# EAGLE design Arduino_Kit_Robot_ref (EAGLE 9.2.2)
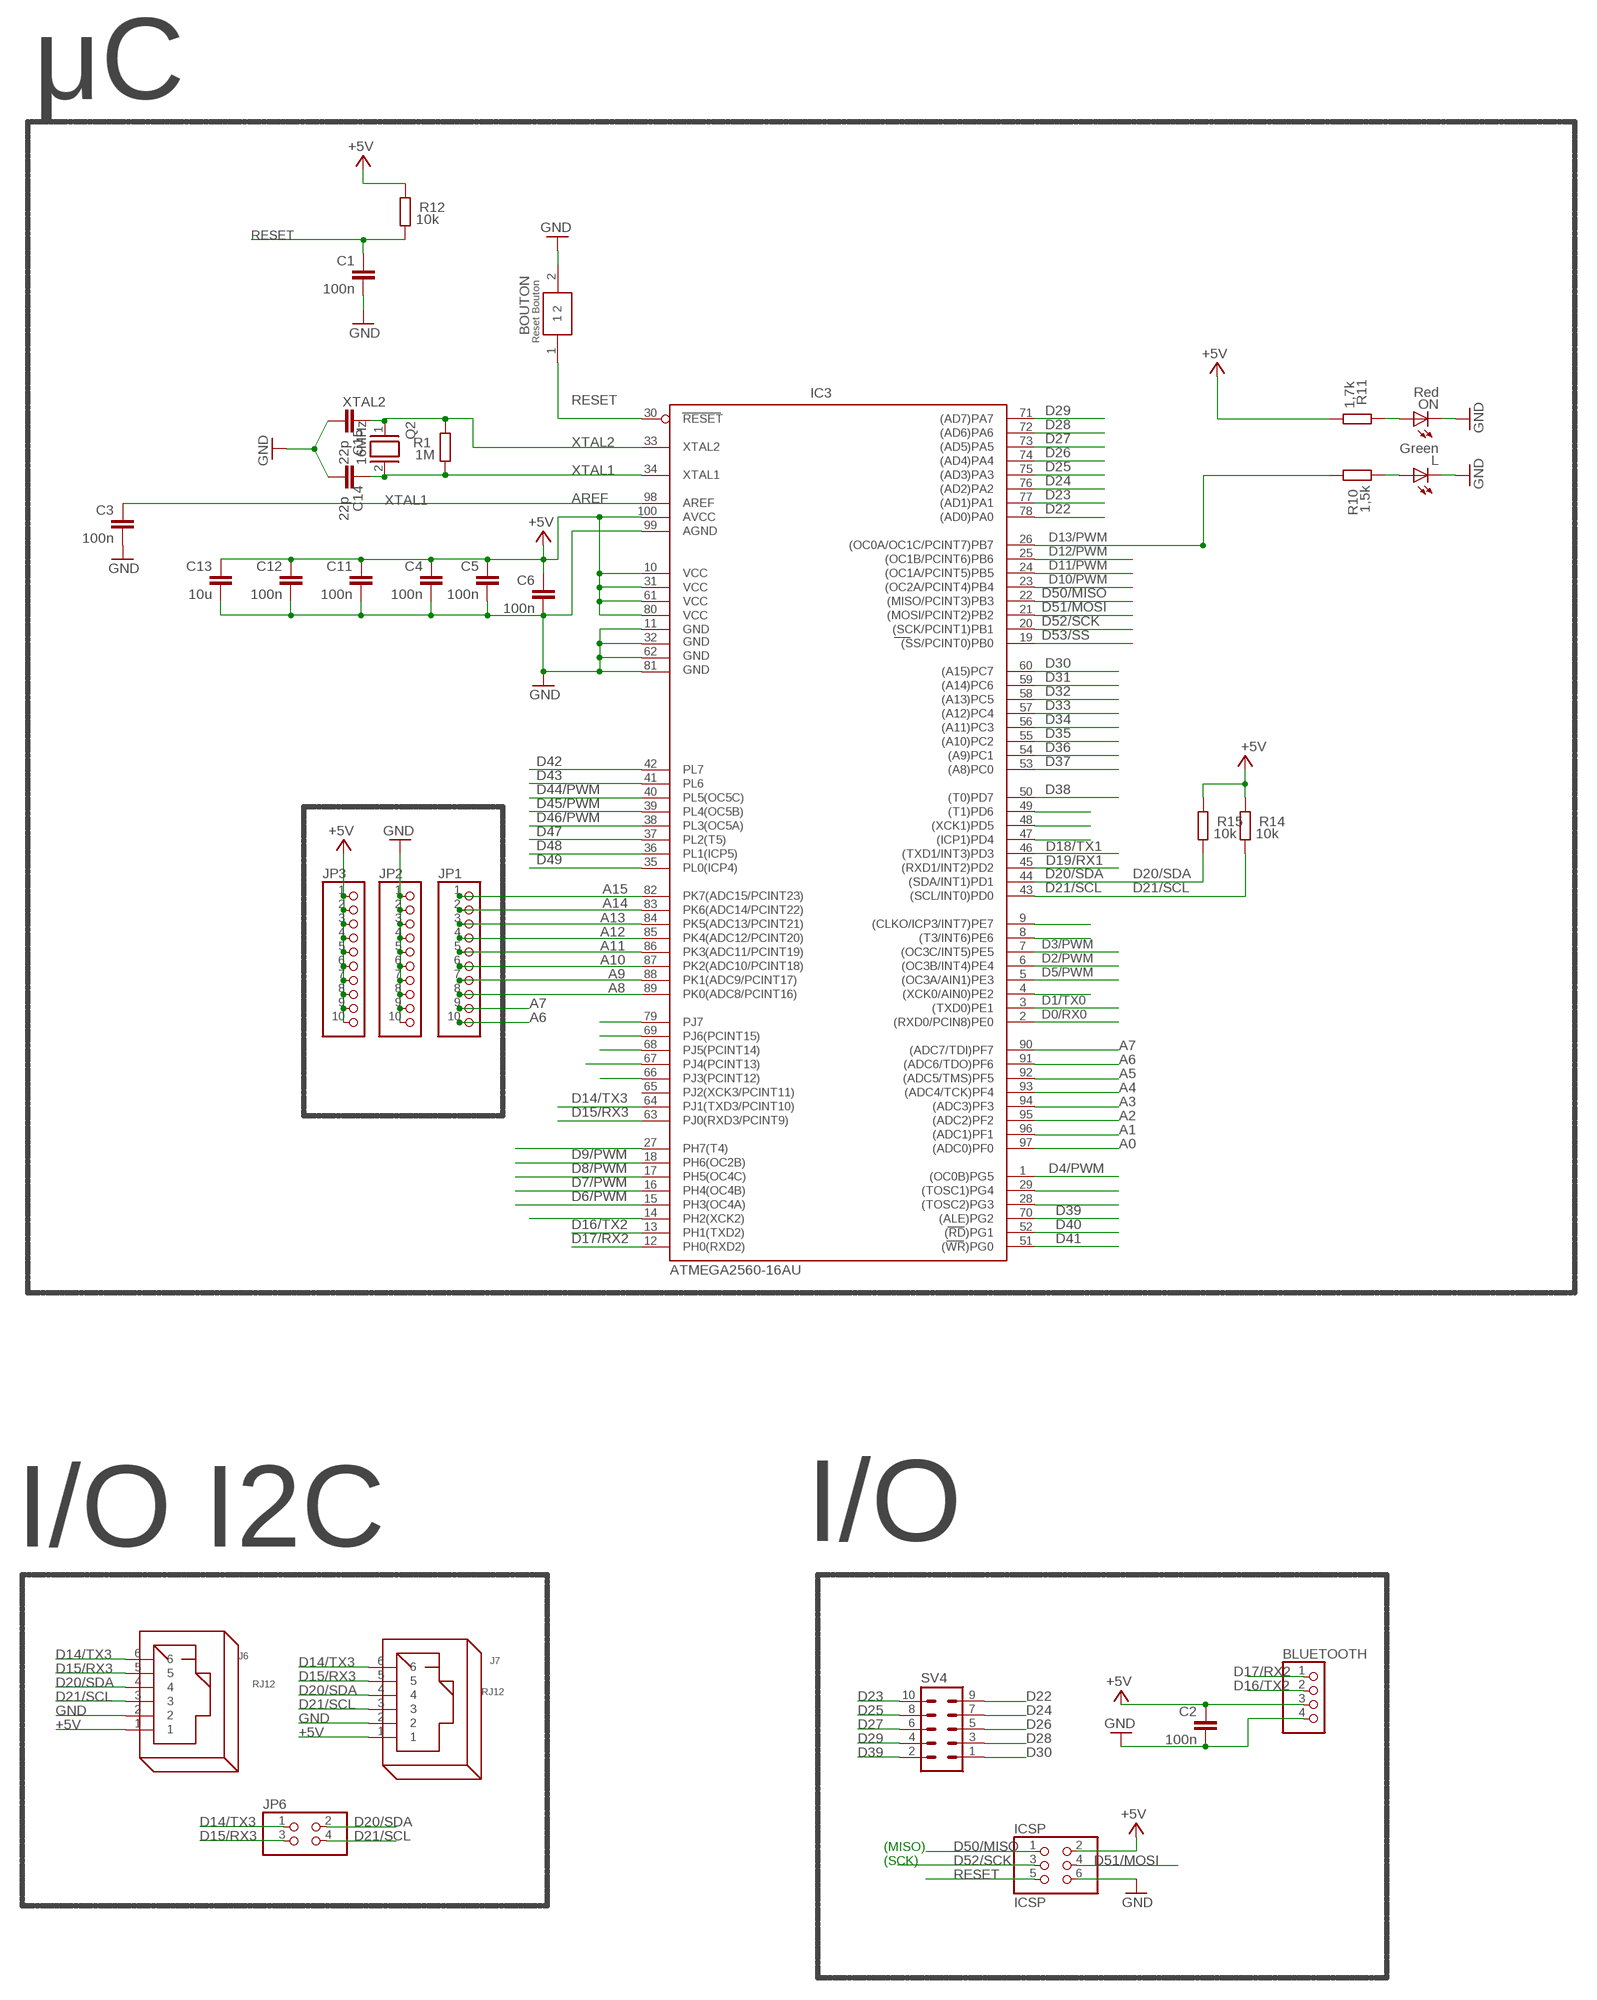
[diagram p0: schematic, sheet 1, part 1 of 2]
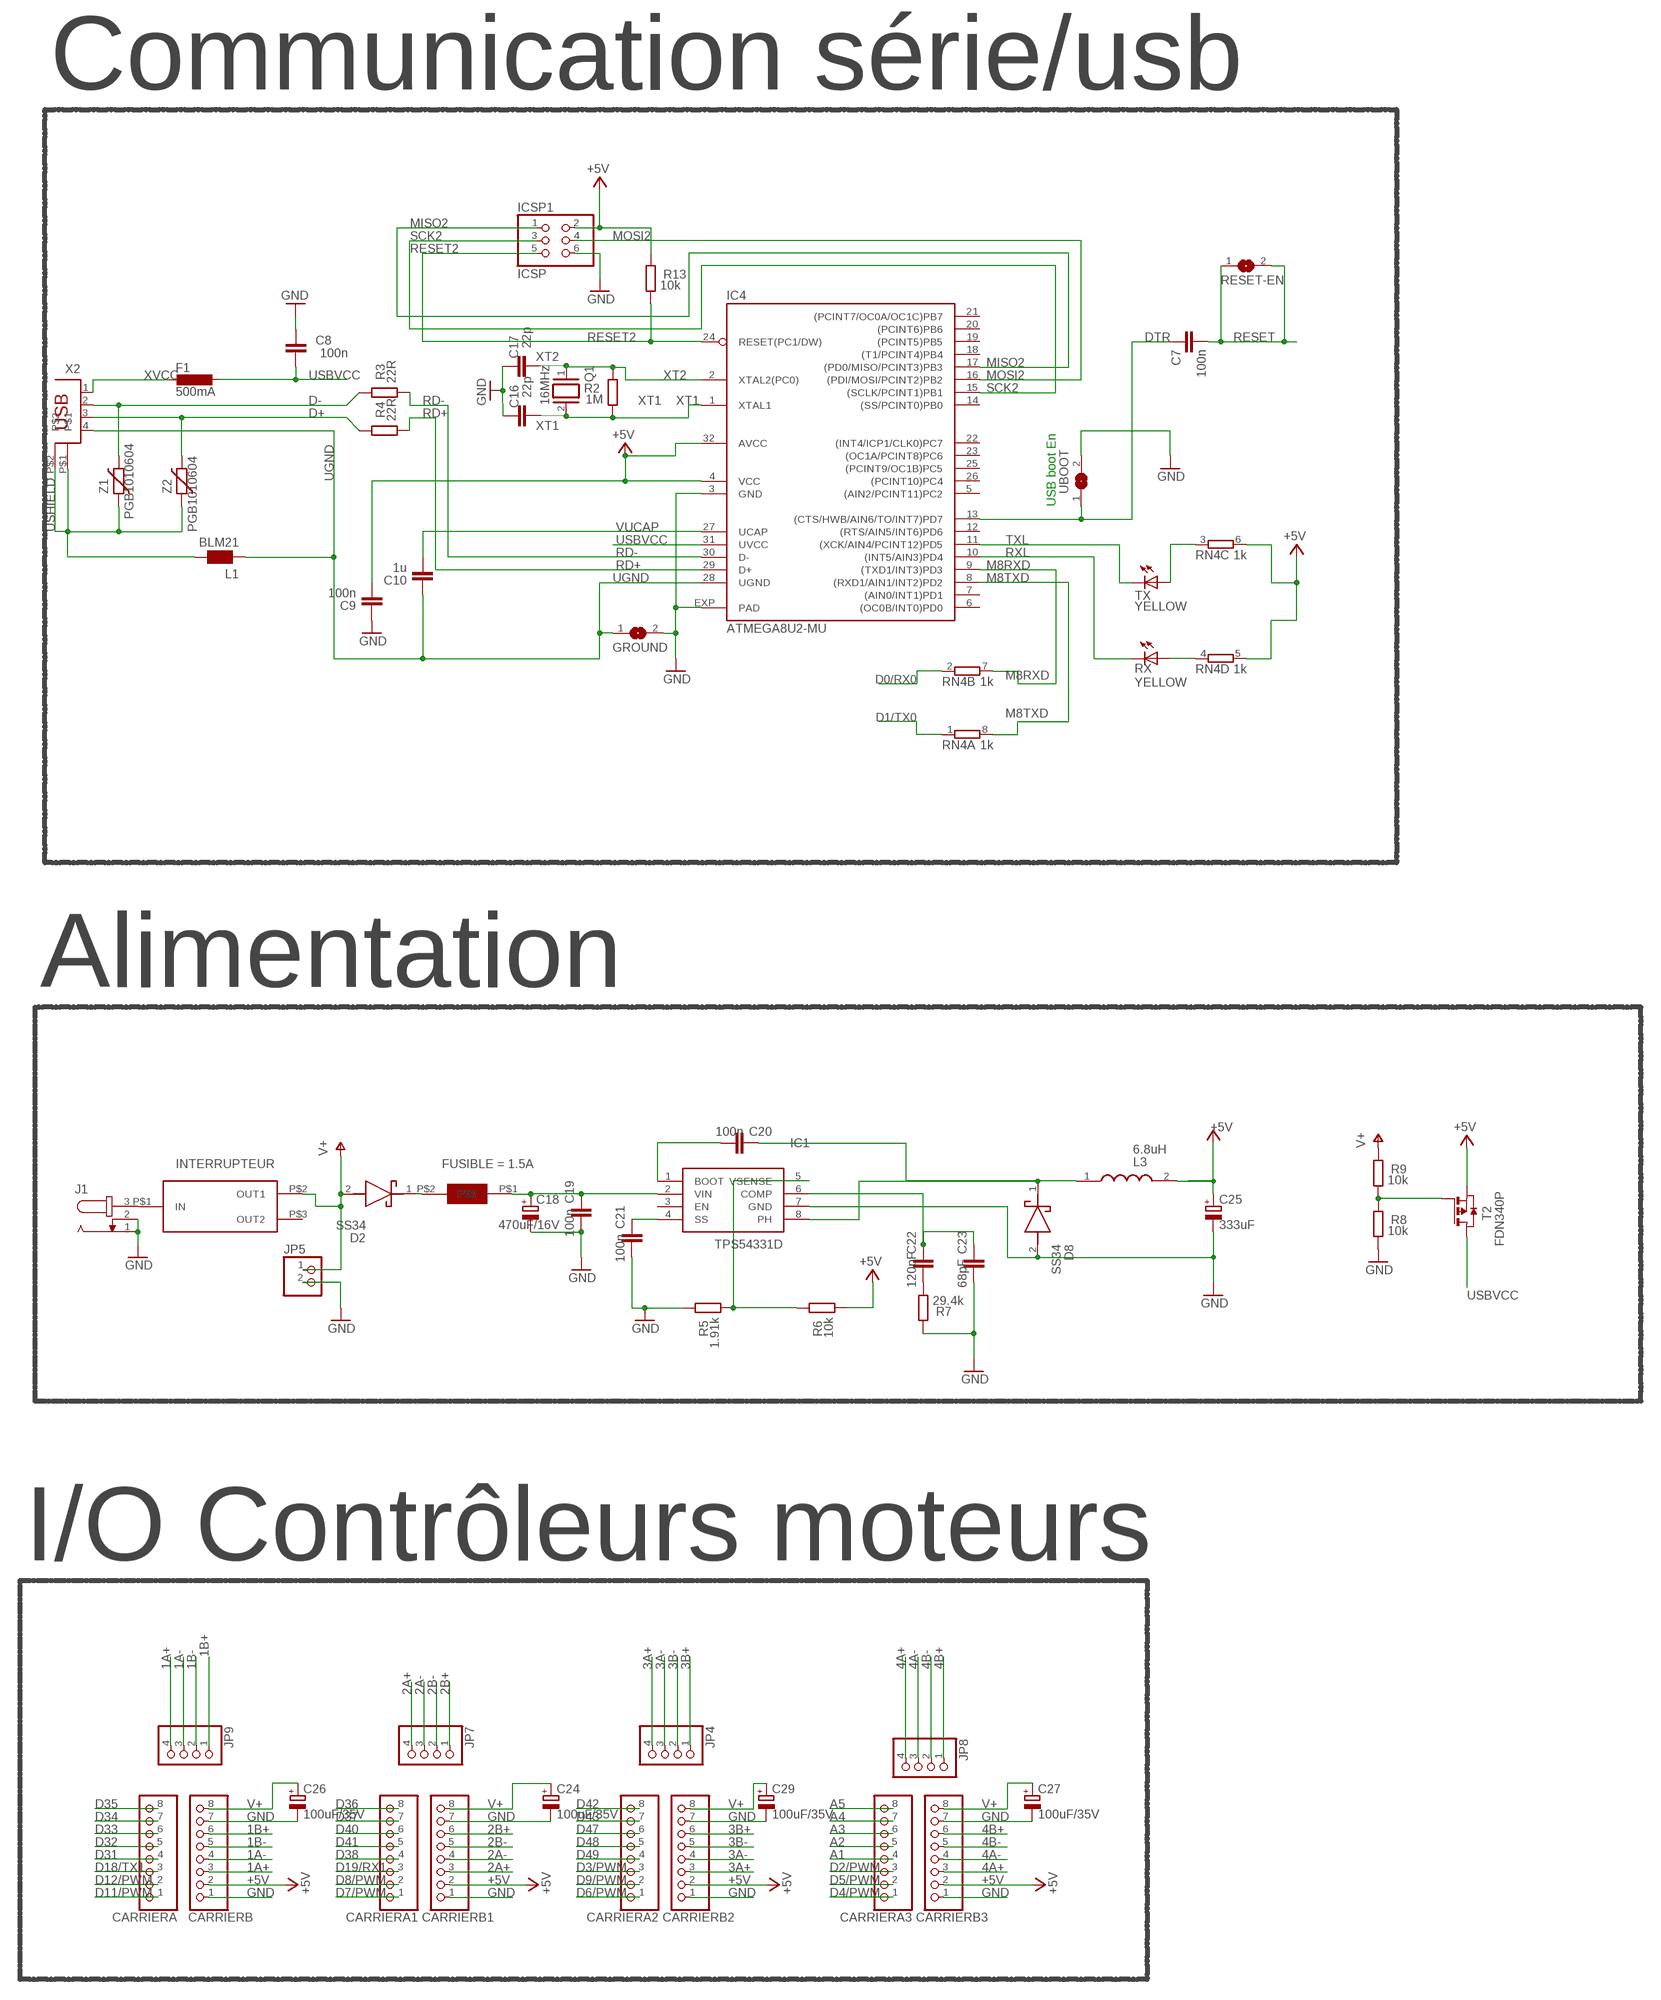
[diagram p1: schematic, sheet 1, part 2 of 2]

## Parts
BLUETOOTH  PINHD-1X4  [1X04]
BOUTON  BOUTON_RESET  [BOUTON_RESET]
C1  100n  C-EU0603-RND  [C0603-ROUND]
C2  100n  C-EU0603-RND  [C0603-ROUND]
C3  100n  C-EU0603-RND  [C0603-ROUND]
C4  100n  C-EU0603-RND  [C0603-ROUND]
C5  100n  C-EU0603-RND  [C0603-ROUND]
C6  100n  C-EU0603-RND  [C0603-ROUND]
C7  100n  C-EU0603-RND  [C0603-ROUND]
C8  100n  C-EUC0603  [C0603]
C9  100n  C-EU0603-RND  [C0603-ROUND]
C10  1u  C-EU0603-RND  [C0603-ROUND]
C11  100n  C-EU0603-RND  [C0603-ROUND]
C12  100n  C-EU0603-RND  [C0603-ROUND]
C13  10u  C-EU0603-RND  [C0603-ROUND]
C14  22p  C-EU0603-RND  [C0603-ROUND]
C15  22p  C-EU0603-RND  [C0603-ROUND]
C16  22p  C-EU0603-RND  [C0603-ROUND]
C17  22p  C-EU0603-RND  [C0603-ROUND]
C18  470uF/16V  CPOL-EUF  [PANASONIC_F]
C19  100n  C-EU0603-RND  [C0603-ROUND]
C20  100n  C-EU0603-RND  [C0603-ROUND]
C21  100n  C-EU0603-RND  [C0603-ROUND]
C22  120pF  C-EU0603-RND  [C0603-ROUND]
C23  68pF  C-EU0603-RND  [C0603-ROUND]
C24  100uF/35V  CPOL-EUF  [PANASONIC_F]
C25  333uF  CPOL-EUD  [PANASONIC_D]
C26  100uF/35V  CPOL-EUF  [PANASONIC_F]
C27  100uF/35V  CPOL-EUF  [PANASONIC_F]
C29  100uF/35V  CPOL-EUF  [PANASONIC_F]
CARRIERA  PINHD-1X8  [1X08]
CARRIERA1  PINHD-1X8  [1X08]
CARRIERA2  PINHD-1X8  [1X08]
CARRIERA3  PINHD-1X8  [1X08]
CARRIERB  PINHD-1X8  [1X08]
CARRIERB1  PINHD-1X8  [1X08]
CARRIERB2  PINHD-1X8  [1X08]
CARRIERB3  PINHD-1X8  [1X08]
D2  SS34  [DIOM8059X256N]
D8  SS34  [DIOM8059X256N]
F1  500mA  L-EUL1812  [L1812]
GROUND  SJ  [SJ]
IC1  TPS54331D  [SOIC127P600X175-8N]
IC3  ATMEGA2560-16AU  ATMEGA1280-16AU  [TQFP100]
IC4  ATMEGA8U2-MU  [QFN32]
ICSP  ICSP  PINHD-2X3  [2X03]
ICSP1  ICSP  PINHD-2X3  [2X03]
J1  JACK-PLUG1  [SPC4078]
J6  RJ12  [RJ12]
J7  RJ12  [RJ12]
JP1  PINHD-1X10  [1X10]
JP2  PINHD-1X10  [1X10]
JP3  PINHD-1X10  [1X10]
JP4  PINHD-1X4/90  [1X04/90]
JP5  PINHD-1X2  [1X02]
JP6  PINHD-2X2  [2X02]
JP7  PINHD-1X4/90  [1X04/90]
JP8  PINHD-1X4/90  [1X04/90]
JP9  PINHD-1X4/90  [1X04/90]
L  Green  LEDCHIP-LED0805  [CHIP-LED0805]
L1  BLM21  WE-CBF_0805  [0805]
L3  6.8uH  7447709006  [WE-PD_1260/1245/1280/121054]
ON  Red  LEDCHIP-LED0805  [CHIP-LED0805]
Q1  16MHz  XTAL/S  [QS]
Q2  16MHz  XTAL/S  [QS]
R1  1M  R-EU_R0603  [R0603-ROUND]
R2  1M  R-EU_R0603  [R0603-ROUND]
R3  22R  R-EU_R0603  [R0603-ROUND]
R4  22R  R-EU_R0603  [R0603-ROUND]
R5  1.91k  R-EU_R0603  [R0603-ROUND]
R6  10k  R-EU_R0603  [R0603-ROUND]
R7  29.4k  R-EU_R0603  [R0603-ROUND]
R8  10k  R-EU_R0603  [R0603-ROUND]
R9  10k  R-EU_R0603  [R0603-ROUND]
R10  1,5k  R-EU_R0603  [R0603-ROUND]
R11  1,7k  R-EU_R0603  [R0603-ROUND]
R12  10k  R-EU_R0603  [R0603-ROUND]
R13  10k  R-EU_R0603  [R0603-ROUND]
R14  10k  R-EU_R0603  [R0603-ROUND]
R15  10k  R-EU_R0603  [R0603-ROUND]
RESET-EN  SJ  [SJ]
RN4  1k  4R-NCAY16  [CAY16]
RX  YELLOW  LEDCHIP-LED0805  [CHIP-LED0805]
SV4  MA05-2  [MA05-2]
T2  FDN340P  PMOSSOT23  [SOT-23]
TX  YELLOW  LEDCHIP-LED0805  [CHIP-LED0805]
U$2  SMD-150  [SMDF-150]
U$3  INTERRUPT  [INTERRUPTEUR]
UBOOT  SJ  [SJ]
X2  PN61729  [PN61729]
Z1  PGB1010604  VARISTORCN0603  [CT/CN0603]
Z2  PGB1010604  VARISTORCN0603  [CT/CN0603]

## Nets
1A+: CARRIERB.3 JP9.4
1A-: CARRIERB.4 JP9.3
1B+: CARRIERB.6 JP9.1
1B-: CARRIERB.5 JP9.2
2A+: CARRIERB1.3 JP7.4
2A-: CARRIERB1.4 JP7.3
2B+: CARRIERB1.6 JP7.1
2B-: CARRIERB1.5 JP7.2
3A+: CARRIERB2.3 JP4.4
3A-: CARRIERB2.4 JP4.3
3B+: CARRIERB2.6 JP4.1
3B-: CARRIERB2.5 JP4.2
4A+: CARRIERB3.3 JP8.4
4A-: CARRIERB3.4 JP8.3
4B+: CARRIERB3.6 JP8.1
4B-: CARRIERB3.5 JP8.2
+5V: BLUETOOTH.3 C2.1 C4.1 C5.1 C6.1 C9.1 C11.1 C12.1 C13.1 C25.+ CARRIERB1.2 CARRIERB2.2 CARRIERB3.2 CARRIERB.2 IC3.10(VCC) IC3.31(VCC1) IC3.61(VCC2) IC3.80(VCC3) IC3.100(AVCC) IC4.4(VCC) IC4.32(AVCC) ICSP1.2 ICSP.2 J6.1 J7.1 JP3.1 JP3.2 JP3.3 JP3.4 JP3.5 JP3.6 JP3.7 JP3.8 JP3.9 JP3.10 L3.2 R6.1 R11.1 R12.2 R13.2 R14.2 R15.2 RN4.5 RN4.6 T2.2(S)
A0: IC3.97((ADC0)PF0)
A1: CARRIERA3.4 IC3.96((ADC1)PF1)
A2: CARRIERA3.5 IC3.95((ADC2)PF2)
A3: CARRIERA3.6 IC3.94((ADC3)PF3)
A4: CARRIERA3.7 IC3.93((ADC4/TCK)PF4)
A5: CARRIERA3.8 IC3.92((ADC5/TMS)PF5)
A6: IC3.91((ADC6/TDO)PF6) JP1.10
A7: IC3.90((ADC7/TDI)PF7) JP1.9
A8: IC3.89(PK0(ADC8/PCINT16)) JP1.8
A9: IC3.88(PK1(ADC9/PCINT17)) JP1.7
A10: IC3.87(PK2(ADC10/PCINT18)) JP1.6
A11: IC3.86(PK3(ADC11/PCINT19)) JP1.5
A12: IC3.85(PK4(ADC12/PCINT20)) JP1.4
A13: IC3.84(PK5(ADC13/PCINT21)) JP1.3
A14: IC3.83(PK6(ADC14/PCINT22)) JP1.2
A15: IC3.82(PK7(ADC15/PCINT23)) JP1.1
AREF: C3.1 IC3.98(AREF)
D0/RX0: IC3.2((RXD0/PCIN8)PE0) RN4.2
D1/TX0: IC3.3((TXD0)PE1) RN4.1
D2/PWM: CARRIERA3.3 IC3.6((OC3B/INT4)PE4)
D3/PWM: CARRIERA2.3 IC3.7((OC3C/INT5)PE5)
D4/PWM: CARRIERA3.1 IC3.1((OC0B)PG5)
D5/PWM: CARRIERA3.2 IC3.5((OC3A/AIN1)PE3)
D6/PWM: CARRIERA2.1 IC3.15(PH3(OC4A))
D7/PWM: CARRIERA1.1 IC3.16(PH4(OC4B))
D8/PWM: CARRIERA1.2 IC3.17(PH5(OC4C))
D9/PWM: CARRIERA2.2 IC3.18(PH6(OC2B))
D10/PWM: IC3.23((OC2A/PCINT4)PB4)
D11/PWM: CARRIERA.1 IC3.24((OC1A/PCINT5)PB5)
D12/PWM: CARRIERA.2 IC3.25((OC1B/PCINT6)PB6)
D13/PWM: IC3.26((OC0A/OC1C/PCINT7)PB7) R10.2
D14/TX3: IC3.64(PJ1(TXD3/PCINT10)) J6.6 J7.6 JP6.1
D15/RX3: IC3.63(PJ0(RXD3/PCINT9)) J6.5 J7.5 JP6.3
D16/TX2: BLUETOOTH.2 IC3.13(PH1(TXD2))
D17/RX2: BLUETOOTH.1 IC3.12(PH0(RXD2))
D18/TX1: CARRIERA.3 IC3.46((TXD1/INT3)PD3)
D19/RX1: CARRIERA1.3 IC3.45((RXD1/INT2)PD2)
D20/SDA: IC3.44((SDA/INT1)PD1) J6.4 J7.4 JP6.2 R15.1
D21/SCL: IC3.43((SCL/INT0)PD0) J6.3 J7.3 JP6.4 R14.1
D22: IC3.78((AD0)PA0) SV4.9
D23: IC3.77((AD1)PA1) SV4.10
D24: IC3.76((AD2)PA2) SV4.7
D25: IC3.75((AD3)PA3) SV4.8
D26: IC3.74((AD4)PA4) SV4.5
D27: IC3.73((AD5)PA5) SV4.6
D28: IC3.72((AD6)PA6) SV4.3
D29: IC3.71((AD7)PA7) SV4.4
D30: IC3.60((A15)PC7) SV4.1
D31: CARRIERA.4 IC3.59((A14)PC6)
D32: CARRIERA.5 IC3.58((A13)PC5)
D33: CARRIERA.6 IC3.57((A12)PC4)
D34: CARRIERA.7 IC3.56((A11)PC3)
D35: CARRIERA.8 IC3.55((A10)PC2)
D36: CARRIERA1.8 IC3.54((A9)PC1)
D37: CARRIERA1.7 IC3.53((A8)PC0)
D38: CARRIERA1.4 IC3.50((T0)PD7)
D39: IC3.70((ALE)PG2) SV4.2
D40: CARRIERA1.6 IC3.52((RD)PG1)
D41: CARRIERA1.5 IC3.51((WR)PG0)
D42: CARRIERA2.8 IC3.42(PL7)
D43: CARRIERA2.7 IC3.41(PL6)
D44/PWM: IC3.40(PL5(OC5C))
D45/PWM: IC3.39(PL4(OC5B))
D46/PWM: IC3.38(PL3(OC5A))
D47: CARRIERA2.6 IC3.37(PL2(T5))
D48: CARRIERA2.5 IC3.36(PL1(ICP5))
D49: CARRIERA2.4 IC3.35(PL0(ICP4))
D50/MISO: IC3.22((MISO/PCINT3)PB3) ICSP.1
D51/MOSI: IC3.21((MOSI/PCINT2)PB2) ICSP.4
D52/SCK: IC3.20((SCK/PCINT1)PB1) ICSP.3
D53/SS: IC3.19((SS/PCINT0)PB0)
D+: R4.2 X2.3 Z2.2
D-: R3.2 X2.2 Z1.2
DTR: C7.1 IC4.13((CTS/HWB/AIN6/TO/INT7)PD7) UBOOT.1
GND: BLUETOOTH.4 BOUTON.2 C1.2 C2.2 C3.2 C4.2 C5.2 C6.2 C8.2 C9.2 C11.2 C12.2 C13.2 C14.1 C15.1 C16.2 C17.2 C18.- C19.1 C21.1 C23.1 C24.- C25.- C26.- C27.- C29.- CARRIERB1.1 CARRIERB1.7 CARRIERB2.1 CARRIERB2.7 CARRIERB3.1 CARRIERB3.7 CARRIERB.1 CARRIERB.7 D8.2(A) GROUND.2 IC1.7(GND) IC3.11(GND) IC3.32(GND1) IC3.62(GND2) IC3.81(GND3) IC3.99(AGND) IC4.3(GND) IC4.EXP(PAD) ICSP1.6 ICSP.6 J1.1 J1.2 J6.2 J7.2 JP2.1 JP2.2 JP2.3 JP2.4 JP2.5 JP2.6 JP2.7 JP2.8 JP2.9 JP2.10 JP5.2 L.C ON.C R5.2 R7.2 R8.1 UBOOT.2
M8RXD: IC4.9((TXD1/INT3)PD3) RN4.7
M8TXD: IC4.8((RXD1/AIN1/INT2)PD2) RN4.8
MISO2: IC4.17((PD0/MISO/PCINT3)PB3) ICSP1.1
MOSI2: IC4.16((PDI/MOSI/PCINT2)PB2) ICSP1.4
N$1: J1.3 U$3.P$1(IN)
N$2: L.A R10.1
N$3: ON.A R11.2
N$4: D2.1(K) U$2.P$2
N$5: C18.+ C19.2 IC1.2(VIN) U$2.P$1
N$6: C20.1 IC1.1(BOOT)
N$7: R8.2 R9.1 T2.3(G)
N$8: C21.2 IC1.4(SS)
N$9: C22.1 R7.1
N$10: IC1.5(VSENSE) R5.1 R6.2
N$11: IC3.49((T1)PD6)
N$12: C22.2 C23.2 IC1.6(COMP)
N$13: C20.2 D8.1(K) IC1.8(PH) L3.1
N$14: IC3.48((XCK1)PD5)
N$15: IC3.47((ICP1)PD4)
N$16: IC3.4((XCK0/AIN0)PE2)
N$17: IC3.9((CLKO/ICP3/INT7)PE7)
N$18: IC3.8((T3/INT6)PE6)
N$19: IC3.29((TOSC1)PG4)
N$20: IC3.28((TOSC2)PG3)
N$21: IC3.27(PH7(T4))
N$22: IC3.14(PH2(XCK2))
N$23: IC3.79(PJ7)
N$24: IC3.69(PJ6(PCINT15))
N$25: IC3.68(PJ5(PCINT14))
N$26: IC3.67(PJ4(PCINT13))
N$27: IC3.66(PJ3(PCINT12))
N$54: RN4.4 RX.A
N$55: RN4.3 TX.A
RD+: IC4.29(D+) R4.1
RD-: IC4.30(D-) R3.1
RESET: BOUTON.1 C1.1 C7.2 IC3.30(RESET) ICSP.5 R12.1 RESET-EN.1 RESET-EN.2
RESET2: IC4.24(RESET(PC1/DW)) ICSP1.5 R13.1
RXL: IC4.10((INT5/AIN3)PD4) RX.C
SCK2: IC4.15((SCLK/PCINT1)PB1) ICSP1.3
TXL: IC4.11((XCK/AIN4/PCINT12)PD5) TX.C
UGND: C10.2 GROUND.1 IC4.28(UGND) L1.1 X2.4
USBVCC: C8.1 F1.1 IC4.31(UVCC) T2.1(D)
USHIELD: L1.2 X2.P$1 X2.P$2 Z1.1 Z2.1
V+: C24.+ C26.+ C27.+ C29.+ CARRIERB1.8 CARRIERB2.8 CARRIERB3.8 CARRIERB.8 D2.2(A) JP5.1 R9.2 U$3.P$2(OUT1)
VUCAP: C10.1 IC4.27(UCAP)
XT1: C16.1 IC4.1(XTAL1) Q1.2 R2.1
XT2: C17.1 IC4.2(XTAL2(PC0)) Q1.1 R2.2
XTAL1: C14.2 IC3.34(XTAL1) Q2.2 R1.1
XTAL2: C15.2 IC3.33(XTAL2) Q2.1 R1.2
XVCC: F1.2 X2.1
Unconnected: IC1.3(EN) IC3.65(PJ2(XCK3/PCINT11)) IC4.5((AIN2/PCINT11)PC2) IC4.6((OC0B/INT0)PD0) IC4.7((AIN0/INT1)PD1) IC4.12((RTS/AIN5/INT6)PD6) IC4.14((SS/PCINT0)PB0) IC4.18((T1/PCINT4)PB4) IC4.19((PCINT5)PB5) IC4.20((PCINT6)PB6) IC4.21((PCINT7/OC0A/OC1C)PB7) IC4.22((INT4/ICP1/CLK0)PC7) IC4.23((OC1A/PCINT8)PC6) IC4.25((PCINT9/OC1B)PC5) IC4.26((PCINT10)PC4) U$3.P$3(OUT2)

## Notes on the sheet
- μC | Communication série/usb
- USB boot En
- Alimentation
- I/O I2C | I/O
- I/O Contrôleurs moteurs
- (MISO)
- (SCK)

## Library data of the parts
BLUETOOTH JP4 JP7-JP9 = pinhead:PINHD-1X4: PIN HEADER
BOUTON = MyLib:BOUTON_RESET
C1-C7 C9-C17 C19-C23 = SmartPrj:C-EU: CAPACITOR, European symbol
C8 = rcl:C-EU: CAPACITOR, European symbol
C18 C24-C27 C29 = rcl:CPOL-EU: POLARIZED CAPACITOR, European symbol; SPICEPREFIX: C
CARRIERA CARRIERA1-CARRIERA3 CARRIERB CARRIERB1-CARRIERB3 = pinhead:PINHD-1X8: PIN HEADER
D2 D8 = SamacSys_Parts:SS34: ON Semi SS34 SMT Schottky Diode, 40V 3A, 2-Pin DO-214AB; DESCRIPTION: ON Semi SS34 SMT Schottky Diode, 40V 3A, 2-Pin DO-214AB; HEIGHT: 2.56mm; MANUFACTURER_NAME: ON Semiconductor; MANUFACTURER_PART_NUMBER: SS34; RS_PART_NUMBER: 1662321
F1 = rcl:L-EU: INDUCTOR, European symbol
GROUND RESET-EN UBOOT = jumper:SJ: SMD solder JUMPER
IC1 = SamacSys_Parts:TPS54331D: Texas Instruments, TPS54331D Step-Down Switching Regulator 3A Adjustable, Minimum of 0.8 V, 8-Pin SOIC Source: Datasheet; DESCRIPTION: Texas Instruments, TPS54331D Step-Down Switching Regulator 3A Adjustable, Minimum of 0.8 V, 8-Pin SOIC; HEIGHT: mm; MANUFACTURER_NAME: Texas Instruments; MANUFACTURER_PART_NUMBER: TPS54331D; RS_PART_NUMBER: 6618521P; RS_PRICE-STOCK: http://uk.rs-online.com/web/p/products/6618521P
IC3 = atmel-2005:ATMEGA*: MICROCONTROLLER 64/128/256 Kbytes FLASH 4 Kbytes EEPROM 8 Kbytes SRAM 86 General Purpose I/O pins 12-channels16-bit PWM 4 x Serial USARTs 16-channels 10-bit A/D
IC4 = atmel:ATMEGA8U2-MU
ICSP ICSP1 = pinhead:PINHD-2X3: PIN HEADER
J1 = con-jack:JACK-PLUG: DC POWER JACK Power Jack, DC, Right Angle, Through Hole, Rated 5A at 16VDC, PC Terminals Distributor: Farnell (www.Farnell.de) Drawing: 84N1161.pdf / 84N1162.pdf Manufacturer: SPC Technology (www.spctechnology.com) Type: SPC4077 / SPC 4078; OC_FARNELL: unknown; OC_NEWARK: unknown
J6 J7 = con-rj:RJ12: RJ12, RJ14 and RJ25 RJ12, RJ14 and RJ25 jacks side mounted http://www.tycoelectronics.com
JP1-JP3 = pinhead:PINHD-1X10: PIN HEADER
JP5 = pinhead:PINHD-1X2: PIN HEADER
JP6 = pinhead:PINHD-2X2: PIN HEADER
L ON RX TX = led:LED: LED
L1 = wuerth-elektronik:WE-CBF: SMD EMI Suppression Ferrite Beads
L3 = SamacSys_Parts:7447709006: Wurth WE-PD Series Shielded Wire-wound SMD Inductor 6.8 uH +/-20% 8.4A Idc; DESCRIPTION: Wurth WE-PD Series Shielded Wire-wound SMD Inductor 6.8 uH +/-20% 8.4A Idc; HEIGHT: mm; MANUFACTURER_NAME: Wurth Elektronik; MANUFACTURER_PART_NUMBER: 7447709006; RS_PART_NUMBER: 7896776; RS_PRICE-STOCK: http://uk.rs-online.com/web/p/products/7896776
Q1 Q2 = special:XTAL/S: CRYSTAL
R1-R15 = SmartPrj:R-EU_: RESISTOR, European symbol
RN4 = resistor-dil:4R-N: Array Chip Resistor Source: RS Component / Phycomp
SV4 = con-lstb:MA05-2: PIN HEADER; OC_FARNELL: unknown; OC_NEWARK: unknown
T2 = zetex:PMOSSOT23: MOS FET
U$2 = MyLib:SMD-150; FUSIBLE: 1.5A
U$3 = MyLib:INTERRUPT
X2 = SmartPrj:PN61729: BERG USB connector
Z1 Z2 = varistor:VARISTOR: VARISTOR

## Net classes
0 default: width 0.15 mm, drill 0.3 mm, clearance 0.15 mm

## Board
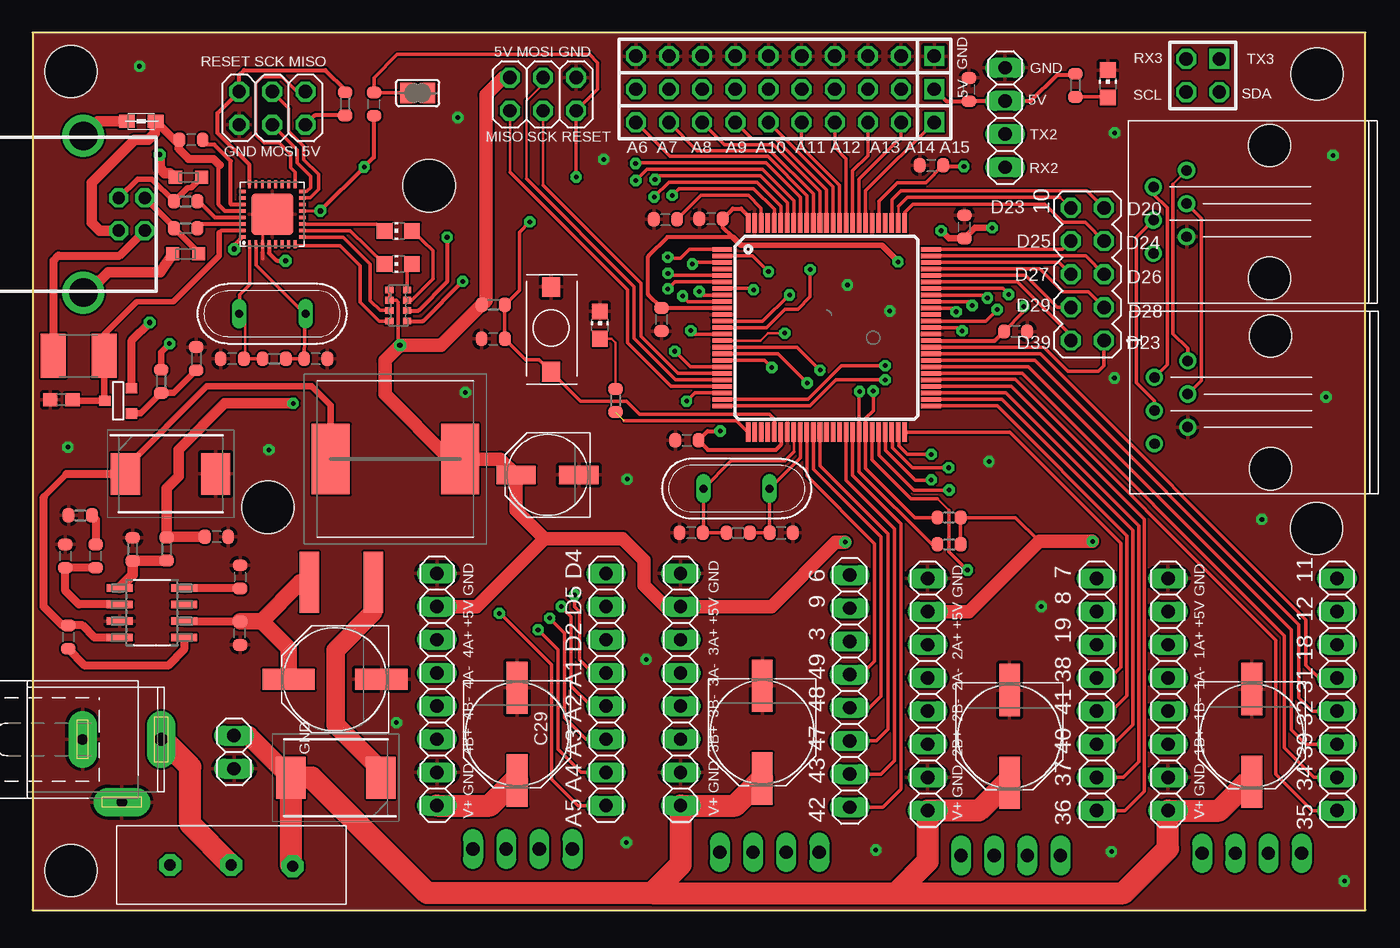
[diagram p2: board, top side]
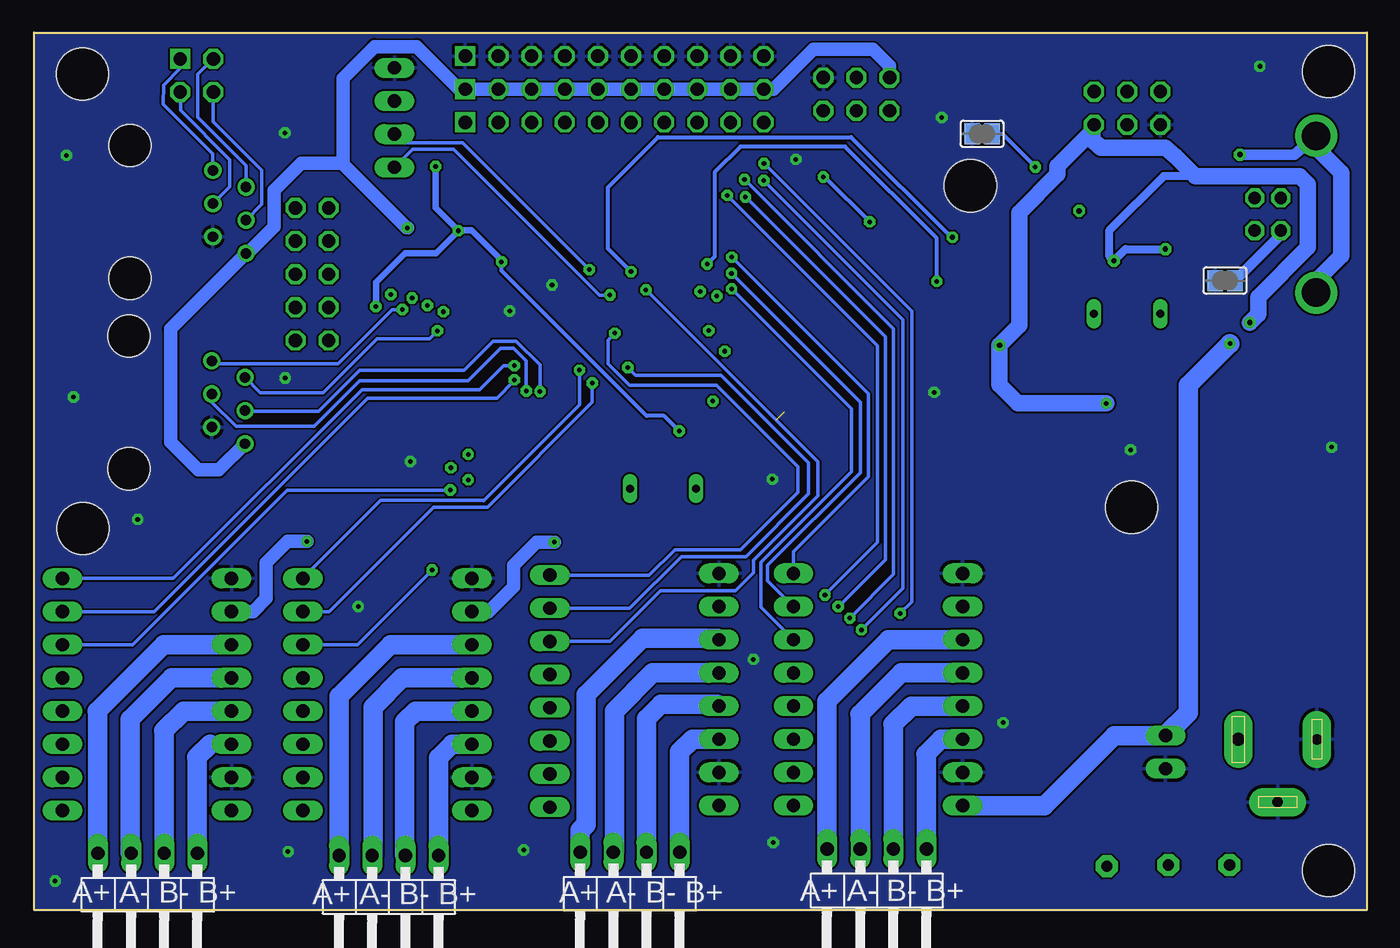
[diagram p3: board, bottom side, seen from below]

Size 102.1 x 67.2 mm. Coordinates in mm from the lower left corner, seen from the top.
Outline: 102.1,0 102.1,67.2 0,67.2 0,0 102.1,0
Copper layers (1*16): Top 0.035mm / dielectric 1.5mm / Bottom 0.035mm
Design rules "default *": minimum track width 0.15mm, minimum drill 0.3mm, track to track 0.15mm, track to pad 0.15mm, pad to pad 0.15mm, via to via 0.15mm, smd to smd 0.15mm, copper to edge 0mil, drill to drill 0.3mm, minimum pad ring 10mil, minimum via ring 10mil, stop-mask expansion 2mil, vias tented up to drill 1mil, thermal gap 10mil
Holes 4 mm at 18.02,30.85 30.38,55.48 2.93,64.23 2.95,3.02 98.35,29.22 98.4,64.03

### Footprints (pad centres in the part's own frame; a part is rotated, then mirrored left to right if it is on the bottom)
1X04 = drill 1.016 long: 1 -3.81,0; 2 -1.27,0; 3 1.27,0; 4 3.81,0
BOUTON_RESET = smd 1.5 x 1.4: 1 0.752,0.7; 2 7.249,0.702
C0603-ROUND = smd 0.898 x 1.1: 1 -0.889,0; 2 0.889,0
C0603 = smd 1.1 x 1: 1 -0.85,0; 2 0.85,0
PANASONIC_F = smd 4 x 1.6: + 3.55,0; - -3.55,0
PANASONIC_D = smd 3 x 1.4: + 2.4,0; - -2.4,0
1X08 = drill 1.016 long: 1 -8.89,0; 2 -6.35,0; 3 -3.81,0; 4 -1.27,0; 5 1.27,0; 6 3.81,0; 7 6.35,0; 8 8.89,0
DIOM8059X256N = smd 2.25 x 3.2: 1 -3.45,0; 2 3.45,0
L1812 = smd 1.9 x 3.4: 1 -1.95,0; 2 1.95,0
SJ = smd 1.168 x 1.6: 1 -0.762,0; 2 0.762,0
SOIC127P600X175-8N = smd 1.981 x 0.559: 1 -2.464,1.905; 2 -2.464,0.635; 3 -2.464,-0.635; 4 -2.464,-1.905; 5 2.464,-1.905; 6 2.464,-0.635; 7 2.464,0.635; 8 2.464,1.905
TQFP100 = smd 1.5 x 0.35: 1 -8,6; 2 -8,5.5; 3 -8,5; 4 -8,4.5; 5 -8,4; 6 -8,3.5; 7 -8,3; 8 -8,2.5; 9 -8,2; 10 -8,1.5; 11 -8,1; 12 -8,0.5; 13 -8,0; 14 -8,-0.5; 15 -8,-1; 16 -8,-1.5; 17 -8,-2; 18 -8,-2.5; 19 -8,-3; 20 -8,-3.5; 21 -8,-4; 22 -8,-4.5; 23 -8,-5; 24 -8,-5.5; 25 -8,-6; 51 8,-6; 52 8,-5.5; 53 8,-5; 54 8,-4.5; 55 8,-4; 56 8,-3.5; 57 8,-3; 58 8,-2.5; 59 8,-2; 60 8,-1.5; 61 8,-1; 62 8,-0.5; 63 8,0; 64 8,0.5; 65 8,1; 66 8,1.5; 67 8,2; 68 8,2.5; 69 8,3; 70 8,3.5; 71 8,4; 72 8,4.5; 73 8,5; 74 8,5.5; 75 8,6 | smd 0.35 x 1.5: 26 -6,-8; 27 -5.5,-8; 28 -5,-8; 29 -4.5,-8; 30 -4,-8; 31 -3.5,-8; 32 -3,-8; 33 -2.5,-8; 34 -2,-8; 35 -1.5,-8; 36 -1,-8; 37 -0.5,-8; 38 0,-8; 39 0.5,-8; 40 1,-8; 41 1.5,-8; 42 2,-8; 43 2.5,-8; 44 3,-8; 45 3.5,-8; 46 4,-8; 47 4.5,-8; 48 5,-8; 49 5.5,-8; 50 6,-8; 76 6,8; 77 5.5,8; 78 5,8; 79 4.5,8; 80 4,8; 81 3.5,8; 82 3,8; 83 2.5,8; 84 2,8; 85 1.5,8; 86 1,8; 87 0.5,8; 88 0,8; 89 -0.5,8; 90 -1,8; 91 -1.5,8; 92 -2,8; 93 -2.5,8; 94 -3,8; 95 -3.5,8; 96 -4,8; 97 -4.5,8; 98 -5,8; 99 -5.5,8; 100 -6,8
QFN32 = smd 0.6 x 0.3: 1 -2.3,1.75; 2 -2.3,1.25; 3 -2.3,0.75; 4 -2.3,0.25; 5 -2.3,-0.25; 6 -2.3,-0.75; 7 -2.3,-1.25; 8 -2.3,-1.75; 17 2.3,-1.75; 18 2.3,-1.25; 19 2.3,-0.75; 20 2.3,-0.25; 21 2.3,0.25; 22 2.3,0.75; 23 2.3,1.25; 24 2.3,1.75 | smd 0.3 x 0.6: 9 -1.75,-2.3; 10 -1.25,-2.3; 11 -0.75,-2.3; 12 -0.25,-2.3; 13 0.25,-2.3; 14 0.75,-2.3; 15 1.25,-2.3; 16 1.75,-2.3; 25 1.75,2.3; 26 1.25,2.3; 27 0.75,2.3; 28 0.25,2.3; 29 -0.25,2.3; 30 -0.75,2.3; 31 -1.25,2.3; 32 -1.75,2.3 | smd 3.2 x 3.2: EXP 0,0
2X03 = drill 1.016 octagon: 1 -2.54,-1.27; 2 -2.54,1.27; 3 0,-1.27; 4 0,1.27; 5 2.54,-1.27; 6 2.54,1.27
SPC4078 = drill 0.8 pad 2.184 long: 1 -3,0; 2 0,-4.8 | drill 1 pad 2.184 long: 3 3,0
RJ12 = drill 0.8: 1 -8.89,-3.175; 2 -6.35,-1.905; 3 -8.89,-0.635; 4 -6.35,0.635; 5 -8.89,1.905; 6 -6.35,3.175 | hole 3.25: 0,-5.08; 0,5.08
1X10 = drill 1.016 square: 1 -11.43,0 | drill 1.016 octagon: 2 -8.89,0; 3 -6.35,0; 4 -3.81,0; 5 -1.27,0; 6 1.27,0; 7 3.81,0; 8 6.35,0; 9 8.89,0; 10 11.43,0
1X04/90 = drill 1.016 long: 1 -3.81,-3.81; 2 -1.27,-3.81; 3 1.27,-3.81; 4 3.81,-3.81
1X02 = drill 1.016 long: 1 -1.27,0; 2 1.27,0
2X02 = drill 1.016 square: 1 -1.27,-1.27 | drill 1.016 octagon: 2 -1.27,1.27; 3 1.27,-1.27; 4 1.27,1.27
CHIP-LED0805 = smd 1.2 x 1.2: A 0,-1.05; C 0,1.05
0805 = smd 1.2 x 1: 1 -1.1,0; 2 1.1,0
WE-PD_1260/1245/1280/121054 = smd 2.9 x 5.4: 1 -4.95,0; 2 4.95,0
QS = drill 0.61 long: 1 -2.54,0; 2 2.54,0
R0603-ROUND = smd 0.898 x 1.1: 1 -0.889,0; 2 0.889,0
CAY16 = smd 0.5 x 0.65: 1 -1.2,-0.675; 2 -0.4,-0.675; 3 0.4,-0.675; 4 1.2,-0.675; 5 1.2,0.675; 6 0.4,0.675; 7 -0.4,0.675; 8 -1.2,0.675
MA05-2 = drill 1.016 octagon: 1 -5.08,-1.27; 2 -5.08,1.27; 3 -2.54,-1.27; 4 -2.54,1.27; 5 0,-1.27; 6 0,1.27; 7 2.54,-1.27; 8 2.54,1.27; 9 5.08,-1.27; 10 5.08,1.27
SOT-23 = smd 0.787 x 0.889: 1 0.025,-1.016; 2 -0.94,1.016; 3 0.991,1.016
SMDF-150 = smd 1.5 x 4.65: P$1 -2.4,0; P$2 2.5,0
INTERRUPTEUR = drill 0.85 pad 1.676 octagon: P$1 0,0; P$2 -4.7,0.1 | drill 0.9 pad 1.676 octagon: P$3 4.7,0
PN61729 = drill 0.95 octagon: 1 1.25,4.71; 2 -1.25,4.71; 3 -1.25,2.71; 4 1.25,2.71 | drill 2.2: P$1 -6,0; P$2 6,0
CT/CN0603 = smd 1 x 1: 1 -1,0; 2 1,0

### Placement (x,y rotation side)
BLUETOOTH  74.51,60.7 90 top
BOUTON  40.42,40.48 90 top
C1  35.28,43.75 180 top
C2  71.74,62.84 90 top
C3  48.48,52.89 180 top
C4  48.18,45.23 270 top
C5  75.32,44.31 0 top
C6  68.86,57.03 180 top
C7  26.15,61.72 90 top
C8  2.2,39.08 180 top
C9  14.09,28.58 0 top
C10  12.14,59 180 top
C11  50.12,35.98 180 top
C12  51.98,52.95 180 top
C13  71.38,52.32 90 top
C14  57.35,28.89 180 top
C15  50.45,28.89 0 top
C16  15.29,42.22 180 top
C17  21.69,42.22 0 top
C18  23.17,17.67 180 top
C19  15.88,21.2 90 top
C20  2.72,20.91 90 top
C21  15.88,25.52 270 top
C22  4.83,27.11 270 top
C23  2.51,27.11 270 top
C24  55.9,13.62 270 top
C25  39.45,33.33 180 top
C26  74.85,13.3 270 top
C27  93.4,13.38 270 top
C29  37.12,13.47 270 top
CARRIERA  99.94,16.51 270 top
CARRIERA1  81.52,16.51 270 top
CARRIERA2  62.6,16.77 270 top
CARRIERA3  43.93,16.89 270 top
CARRIERB  86.98,16.51 270 top
CARRIERB1  68.57,16.51 270 top
CARRIERB2  49.64,16.89 270 top
CARRIERB3  30.98,16.89 270 top
D2  23.23,10.14 180 top
D8  10.57,33.4 0 top
F1  3.53,42.46 180 top
GROUND  10.87,48.21 180 bottom
IC1  9.14,22.77 180 top
IC3  60.82,44.61 0 top
IC4  18.36,53.29 90 top
ICSP  39.1,62.49 0 top
ICSP1  18.36,61.42 180 top
J1  6.83,13.07 0 top
J6  94.76,53.47 0 top
J7  94.84,38.89 0 top
JP1  57.65,60.33 180 top
JP2  57.65,65.41 180 top
JP3  57.65,62.87 180 top
JP4  56.46,0.62 180 bottom
JP5  15.43,12.1 270 top
JP6  89.65,63.92 180 top
JP7  74.94,0.37 180 bottom
JP8  37.54,0.87 180 bottom
JP9  93.41,0.54 180 bottom
L  43.46,44.8 0 top
L1  8.33,60.4 180 top
L3  27.8,34.55 0 top
ON  82.38,63.29 0 top
Q1  18.36,45.67 180 top
Q2  53.93,32.28 0 top
R1  54.04,28.88 180 top
R2  18.52,42.22 0 top
R3  11.72,52.23 180 top
R4  11.72,54.27 180 top
R5  7.67,27.62 90 top
R6  10.28,27.65 270 top
R7  3.65,30.22 180 top
R8  12.55,42.23 270 top
R9  9.85,40.49 90 top
R10  44.67,39.03 270 top
R11  79.89,63.16 270 top
R12  35.29,46.36 180 top
R13  23.94,61.75 270 top
R14  70.21,28 0 top
R15  70.2,30.07 0 top
RESET-EN  29.5,62.58 0 top
RN4  28.02,46.3 90 top
RX  28.02,49.48 90 top
SV4  80.82,48.7 90 top
T2  6.55,39.03 270 top
TX  28.02,52.02 90 top
U$2  23.6,25.1 0 top
U$3  15.22,3.45 180 top
UBOOT  29.48,59.45 180 bottom
X2  3.89,53.29 270 top
Z1  11.72,50.25 0 top
Z2  11.94,56.13 0 top

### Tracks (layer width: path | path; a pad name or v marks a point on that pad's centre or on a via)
1A+
  Bottom 1.016: 97.22,15.19 97.27,15.24
  Bottom 1.5: 97.27,15.24 92.19,20.32 CARRIERB.3 | JP9.4 97.22,15.19
1A-
  Bottom 1.016: 94.73,4.4 JP9.3
  Bottom 1.5: CARRIERB.4 91.56,17.78 94.73,14.61 94.73,4.4
1B+
  Bottom 1.016: 88.63,12.7 CARRIERB.6 | 89.6,11.64 89.65,11.69
  Bottom 1.5: 89.65,11.69 88.63,12.7 | JP9.1 89.6,11.64
1B-
  Bottom 1.016: 92.14,13.67 92.19,13.72
  Bottom 1.5: CARRIERB.5 90.67,15.24 92.19,13.72 | JP9.2 92.14,13.67
2A+
  Bottom 1.016: JP7.4 78.74,4.19
  Bottom 1.5: CARRIERB1.3 74.79,20.32 78.74,16.38 78.74,4.19
2A-
  Bottom 1.016: JP7.3 76.14,4.24
  Bottom 1.5: CARRIERB1.4 73.9,17.78 76.14,15.54 76.14,4.24
2B+
  Bottom 1.016: JP7.1 71.12,4.19
  Bottom 1.5: CARRIERB1.6 70.09,12.7 71.12,11.68 71.12,4.19
2B-
  Bottom 1.016: JP7.2 73.71,4.22
  Bottom 1.5: CARRIERB1.5 72.89,15.24 73.71,14.42 73.71,4.22
3A+
  Bottom 1.016: 49.77,20.83 CARRIERB2.3
  Bottom 1.5: 49.77,20.83 55.49,20.83 59.84,16.48 59.84,6.54 60.27,6.1 JP4.4
3A-
  Bottom 1.016: 57.65,4.51 JP4.3
  Bottom 1.5: CARRIERB2.4 54.73,18.16 57.65,15.24 57.65,4.51
3B+
  Bottom 1.5: CARRIERB2.6 51.68,13.08 52.65,12.11 JP4.1
3B-
  Bottom 1.016: 49.77,15.75 CARRIERB2.5
  Bottom 1.5: 49.77,15.75 54.09,15.75 55.19,14.65 JP4.2
4A+
  Bottom 1.5: CARRIERB3.3 36.65,20.7 41.35,16 JP8.4
4A-
  Bottom 1.016: 38.81,14.95 38.85,14.99
  Bottom 1.5: 38.85,14.99 35.67,18.16 CARRIERB3.4 | JP8.3 38.81,14.95
4B+
  Bottom 1.016: 33.73,11.9 33.77,11.94
  Bottom 1.5: CARRIERB3.6 32.63,13.08 33.77,11.94 | JP8.1 33.73,11.9
4B-
  Bottom 1.016: 36.27,14.19 36.31,14.23
  Bottom 1.5: CARRIERB3.5 34.91,15.62 36.31,14.23 | JP8.2 36.27,14.19
+5V  (via drill 0.35, 0.41)
  Top 0.203: 48.2,46.1 C4.1 | 71.09,28.01 R14.2
  Top 0.254: v28.14,43.26 28.08,43.38 28.02,43.83 28.02,46.56 27.87,46.7 RN4.6 RN4.5 | C6.1 68.44,55.72 66.26,55.72 64.82,54.29 IC3.80 | 71.09,28.01 R15.2 75.3,30.07 77.12,28.24 | C2.1 71.76,61.97 | 79.81,63.98 R11.1 | 54.82,53.18 IC3.100 | 52.86,52.31 C12.1 | C5.1 75.93,45.81 v75.93,46.23
  Top 0.305: R13.2 21.61,60.86 ICSP1.2 | 36.06,63.76 ICSP.2 | IC3.10 48.2,46.1 | C4.1 47.16,47.14 47.16,50.06 48.64,51.54 53.64,51.54 52.86,52.31 | IC4.4 18.11,50.32 18.7,49.73 v19.38,49.73 | IC4.32 15.44,50.92 | IC3.31 57.32,35.62 56.95,35.25 51.74,35.25 C11.1 51.72,36.68 v52.67,36.68 | 71.76,61.97 BLUETOOTH.3 76.49,61.97 78.5,63.98 79.81,63.98 | IC3.61 73.72,43.6 C5.1 | C12.1 53.64,53.73 54.27,53.73 54.82,53.18 | 69.84,56.95 v71.35,56.95 | JP3.1 69.99,61.95 C2.1
  Top 0.406: 15.44,50.92 v15.44,50.62 | 53.64,51.54 54.27,50.91 65.07,50.91 66.3,49.67 v66.3,49.65
  Top 0.508: v73.51,52.25 72.19,52.25 C13.1 70.19,51.44 v69.6,52.02 | C6.1 69.84,56.95
  Top 0.61: v8.96,45 7.57,43.6 T2.2
  Top 0.813: v19.97,38.81 14.73,38.81 11.18,35.26 11.18,33.22 10.28,32.32 R6.1 10.31,28.58 C9.1
  Top 1.016: 36.06,63.76 34.73,62.43 34.73,46.68 R12.2 34.39,46.36 31.28,43.26 v28.14,43.26 26.99,42.11 26.99,39.51 31.95,34.55 L3.2 35.83,34.55 C25.+ 37.05,30.63 39.23,28.45 | CARRIERB3.2 34.02,23.24 39.23,28.45 | CARRIERB1.2 71.74,22.86 77.12,28.24 v81.2,28.24 | 39.23,28.45 45.2,28.45 46.85,26.8 46.85,24.89 48.5,23.24 CARRIERB2.2 56.59,23.24 61.52,28.17 v62.25,28.17
  Bottom 0.203: 75.73,54.41 75.59,54.28
  Bottom 0.305: v52.67,36.68 53.84,37.85 55.17,37.85 66.3,48.98 v66.3,49.65
  Bottom 0.508: v66.3,49.65 66.3,49.75 68.6,52.05 69.58,52.05 v69.6,52.02 | v75.93,46.23 75.93,48.07 73.7,50.3 71.33,50.3 v69.6,52.02 | v71.35,56.95 71.35,53.77 v69.6,52.02
  Bottom 0.61: 13.16,56.21 15.57,56.21 19.76,52.02 19.76,50.11 v19.38,49.73 18.49,50.62 v15.44,50.62
  Bottom 1.016: ICSP.2 36.56,64.65 37.83,65.92 42.41,65.92 45.45,62.87 JP3.10 JP3.9 JP3.8 JP3.7 JP3.6 JP3.5 JP3.4 JP3.3 JP3.2 JP3.1 69.54,62.87 72.8,66.12 76.03,66.12 78.43,63.72 78.43,57.19 78.5,57.19 | CARRIERB.2 85.33,22.86 84.32,23.88 84.32,26.61 82.69,28.24 v81.2,28.24 | 75.73,54.41 78.5,57.19 | 78.5,57.19 81.65,57.19 83.7,55.13 83.7,52.34 85.75,50.3 J6.1 91.65,44.52 91.65,35.84 89.53,33.71 87.95,33.71 J7.1 | v62.25,28.17 63.6,28.17 65.38,26.4 65.38,24.77 67.29,22.86 CARRIERB1.2 | v73.51,52.25 73.56,52.25 75.59,54.28
  Bottom 1.27: 21.03,59.64 21.03,59 20.4,58.37 15.44,58.37 14.68,57.73 13.16,56.21 5.16,56.21 4.52,55.57 4.52,50.75 8.33,46.94 8.33,45.63 v8.96,45 | ICSP1.2 21.03,60.02 21.03,59.64 | 21.03,59.64 23.7,56.97 23.7,56.34 26.62,53.42 26.62,44.78 v28.14,43.26 28.14,40.22 26.73,38.81 v19.97,38.81
A1  (via drill 0.35)
  Top 0.254: IC3.96 56.82,53.66 55.23,55.25 49.52,55.25 v49.01,54.74 | CARRIERA3.4 42.91,18.16 41.9,19.18 41.9,22.86 41.52,23.24 v41.52,24.13
  Bottom 0.254: v49.01,54.74 37.49,43.22 37.49,28.16 v41.52,24.13
A2  (via drill 0.35)
  Top 0.203: CARRIERA3.5 43.8,15.75
  Top 0.254: IC3.95 57.32,53.92 55.49,55.75 48.75,55.75 v47.61,54.61 | 43.8,15.75 42.66,15.75 41.26,17.15 41.26,22.48 v40.5,23.24
  Bottom 0.254: v47.61,54.61 36.9,43.9 36.9,26.84 v40.5,23.24
A3  (via drill 0.35)
  Top 0.254: IC3.94 57.82,54.18 55.77,56.24 47.97,56.24 v47.69,55.96 | CARRIERA3.6 42.41,13.08 40.75,14.74 40.75,21.21 v39.61,22.35
  Bottom 0.254: v39.61,22.35 36.26,25.7 36.26,44.53 v47.69,55.96
A4  (via drill 0.35)
  Top 0.254: IC3.93 58.32,54.32 55.91,56.73 47.06,56.73 v46.22,55.88 | CARRIERA3.7 42.02,10.54 40.25,12.32 40.25,19.94 v38.72,21.47
  Bottom 0.254: v38.72,21.47 35.55,24.64 35.55,45.21 v46.22,55.88
A5  (via drill 0.35)
  Top 0.254: IC3.92 58.82,54.58 56.18,57.22 46.19,57.22 v46.19,57.18 | CARRIERA3.8 41.77,8 39.74,10.04 39.74,18.8 35.81,22.73 v35.76,22.73
  Bottom 0.254: v35.76,22.73 34.86,23.63 34.86,45.85 v46.19,57.18
A6
  Top 0.254: IC3.91 59.32,54.72 56.32,57.71 48.83,57.71 JP1.10
A7
  Top 0.254: IC3.90 59.82,54.85 56.5,58.17 50.91,58.17 JP1.9
A8
  Top 0.254: JP1.8 53.02,58.61 56.75,58.61 60.32,55.04 IC3.89
A9
  Top 0.254: JP1.7 55.11,59.06 56.93,59.06 60.82,55.16 IC3.88
A10
  Top 0.254: IC3.87 61.32,55.38 JP1.6
A11
  Top 0.254: IC3.86 61.82,55.52 58.92,58.42 JP1.5
A12
  Top 0.254: JP1.4 61.46,58.42 62.32,57.56 IC3.85
A13
  Top 0.254: JP1.3 64,57.79 62.82,56.61 IC3.84
A14
  Top 0.254: IC3.83 63.32,55.97 66.54,59.18 JP1.2
A15
  Top 0.254: IC3.82 63.82,55.07 JP1.1
AREF
  Top 0.254: IC3.98 55.82,53.75 54.83,54.74 51.22,54.74 C3.1
D0/RX0  (via drill 0.35)
  Top 0.254: IC3.2 55.17,50.1 v56.38,48.9
  Top 0.305: v31.75,51.53 31.75,48.1 29.55,45.9 RN4.2
  Bottom 0.203: 31.84,51.53 v31.75,51.53
  Bottom 0.305: v56.38,48.9 58.18,50.7 58.18,55.34 54.31,59.2 39.51,59.2 31.84,51.53
D1/TX0  (via drill 0.35)
  Top 0.254: IC3.3 50.68,49.6 v50.55,49.48
  Top 0.305: RN4.1 29.9,45.1 v32.95,48.15
  Bottom 0.305: v32.95,48.15 32.95,51.45 39.98,58.48 48,58.48 49.98,56.5 49.98,50.05 v50.55,49.48
D2/PWM  (via drill 0.35)
  Top 0.254: IC3.6 51.52,48.1 49.2,48.1 v48.67,47.58
  Bottom 0.254: CARRIERA3.3 46.41,23.18 46.41,26.63 39.48,33.55 39.48,38.38 v48.67,47.58
D3/PWM  (via drill 0.35)
  Top 0.254: IC3.7 55.13,47.6 v55.23,47.5
  Bottom 0.254: CARRIERA2.3 57.97,20.58 54.11,24.44 48.39,24.44 47,25.82 47.01,26.78 42.05,31.73 42.05,34.32 v55.23,47.5
D4/PWM  (via drill 0.35)
  Top 0.203: v48.66,50 48.75,49.91
  Top 0.254: 48.75,49.91 49.63,49.91 50.32,50.6 IC3.1
  Bottom 0.254: v48.66,50 38.19,39.54 38.19,33.17 43.93,27.43 CARRIERA3.1
D5/PWM  (via drill 0.35)
  Top 0.203: 52.81,48.62 IC3.5
  Top 0.254: 52.81,48.62 48.83,48.62 v48.68,48.77
  Bottom 0.254: CARRIERA3.2 45.91,25.22 45.91,26.39 38.8,33.5 38.8,38.88 48.01,48.09 v48.68,48.77
D6/PWM  (via drill 0.35)
  Top 0.203: IC3.15 55.76,43.6 56.34,44.18 v57.62,44.18
  Bottom 0.254: v57.62,44.18 58.14,43.66 58.14,41.84 56.49,40.18 49.81,40.18 43.59,33.96 43.59,32 47.98,27.6 53.03,27.6 55,25.63 62.57,25.63 CARRIERA2.1
D7/PWM  (via drill 0.35)
  Top 0.254: IC3.16 58.58,43.1 v60.33,41.35
  Bottom 0.203: 67.67,31.36 67.67,31.37
  Bottom 0.254: CARRIERA1.1 75.55,31.37 67.67,31.37 | v60.33,41.35 60.33,38.7 67.67,31.36
D8/PWM  (via drill 0.35)
  Top 0.254: IC3.17 57.1,42.6 v59.35,40.36
  Bottom 0.254: v59.35,40.36 59.35,38.88 67.36,30.86 71.49,30.86 79.49,22.86 CARRIERA1.2
D9/PWM  (via drill 0.35)
  Top 0.254: IC3.18 56.06,42.1 v56.62,41.55
  Bottom 0.254: v56.62,41.55 56.04,40.97 49.47,40.97 42.77,34.27 42.77,31.87 47.57,27.07 52.52,27.07 56.47,23.12 CARRIERA2.2
D10/PWM  (via drill 0.35)
  Top 0.254: IC3.23 50.73,39.6 v50.1,38.98
D11/PWM  (via drill 0.35)
  Top 0.203: IC3.24 52.84,39.12
  Top 0.254: 52.84,39.12 59.39,39.12 61.97,41.69 v65.31,41.69
  Bottom 0.254: v65.31,41.69 66.15,41.69 67.98,39.86 76.99,39.86 91.45,25.4 CARRIERA.1
D12/PWM  (via drill 0.35)
  Top 0.254: IC3.25 59.54,38.6 61.54,40.6 v65.32,40.6
  Bottom 0.254: v65.32,40.6 65.32,40.53 66.65,39.2 76.57,39.2 92.91,22.86 CARRIERA.2
D13/PWM  (1 unrouted)
  Top 0.254: IC3.26 53.94,37.49 45.32,37.49
D14/TX3  (via drill 0.35)
  Top 0.203: J6.6 87.35,55.59
  Top 0.254: IC3.64 73.02,45.1 v73.9,45.99 | 87.35,55.59 87.35,44.15 88.49,43.01 J7.6
  Bottom 0.203: J7.6 88.24,41.82
  Bottom 0.254: v73.9,45.99 74.66,45.99 78.83,41.82 88.24,41.82 | J6.6 88.41,57.94 92.21,61.73 92.2,63.17 90.92,64.45 JP6.1
D15/RX3  (via drill 0.35)
  Top 0.254: v71.22,44.36 70.98,44.6 IC3.63 | J7.5 86.93,41.77 86.93,53.78 85.87,54.83 J6.5
  Bottom 0.254: v71.22,44.36 71.81,43.77 75.82,43.77 79.98,39.62 84.77,39.62 J7.5 | J6.5 85.87,57 89.57,60.7 89.57,64 JP6.3
D16/TX2  (via drill 0.35)
  Top 0.254: IC3.13 56.21,44.6 57.63,46.03 58.62,46.03 59.57,46.99 v59.57,49.05
  Bottom 0.254: BLUETOOTH.2 73.86,58.77 71.75,58.77 69.3,58.77 61.36,50.84 61.24,50.71 v59.57,49.05
D17/RX2  (via drill 0.35)
  Top 0.203: 57.93,47.11 v57.99,47.11
  Top 0.254: IC3.12 55.93,45.1 57.93,47.11
  Bottom 0.254: v57.99,47.11 58.02,47.08 58.78,47.08 69.98,58.27 73.12,58.27 BLUETOOTH.1
D18/TX1  (via drill 0.35)
  Top 0.254: v70.22,32.16 67.52,32.16 64.84,34.84 64.84,36.58
  Top 0.305: 64.84,36.58 IC3.46
  Bottom 0.254: CARRIERA.3 94.55,20.32 82.71,32.16 v70.22,32.16
D19/RX1  (via drill 0.35)
  Top 0.203: 69.34,31.49 70.22,30.61
  Top 0.254: IC3.45 64.32,34.48 67.31,31.49 69.34,31.49 | 70.22,30.61 70.22,27.43 v71.62,26.04
  Bottom 0.254: v71.62,26.04 77.33,20.32 CARRIERA1.3
D20/SDA  (via drill 0.35)
  Top 0.254: R15.1 67.59,30.07 63.82,33.83 IC3.44 63.82,37.67 64.4,38.25 v64.4,39.76 | J7.4 89.53,40.56 89.53,53 J6.4
  Bottom 0.203: JP6.2 90.9,62.62
  Bottom 0.254: J7.4 88.49,38.9 86.64,37.05 80.66,37.05 77.16,40.54 68.86,40.54 66.36,43.04 65.37,43.04 64.4,42.07 v64.4,39.76 | 90.9,62.62 90.9,61.24 87.14,57.48 87.14,55.38 J6.4
D21/SCL  (via drill 0.35)
  Top 0.152: 63.32,39.69 v63.35,39.72
  Top 0.203: R14.1 68.89,28
  Top 0.254: 68.89,28 63.32,33.57 IC3.43 63.32,39.69 | J6.3 84.55,51.52 84.55,40.4 85.95,39 J7.3
  Bottom 0.254: v63.35,39.72 63.35,41.75 65.19,43.58 66.96,43.58 69.18,41.36 77.16,41.36 80.31,38.2 85.9,38.2 J7.3 | J6.3 84.67,54.04 84.67,56.67 88.38,60.38 JP6.4
D22
  Top 0.254: IC3.78 65.82,54.4 66.51,55.09 80.78,55.09 SV4.9
D23
  Top 0.203: IC3.77 66.32,53.91 | SV4.10 78.72,54.61
  Top 0.254: 66.32,53.91 67.02,54.61 78.72,54.61
D24
  Top 0.254: SV4.7 80.66,52.66 78.94,52.66 77.54,54.05 67.45,54.05 66.82,53.43 IC3.76
D25
  Top 0.254: IC3.75 78.91,50.6 SV4.8
D26
  Top 0.254: IC3.74 80.68,50.1 SV4.5
D27
  Top 0.254: IC3.73 78.64,49.6 SV4.6
D28
  Top 0.254: IC3.72 77.18,49.1 78.94,47.34 80.9,47.34 SV4.3
D29
  Top 0.254: IC3.71 76.07,48.6 78.52,46.16 SV4.4
D30
  Top 0.254: IC3.60 77.47,43.1 79.31,41.26 81.64,41.26 82.09,41.7 SV4.1
D31
  Top 0.254: IC3.59 77.19,42.6 97.56,22.24 97.56,18.77 98.54,17.78 CARRIERA.4
D32
  Top 0.254: CARRIERA.5 98.03,15.24 97.02,16.26 97.02,21.86 76.77,42.1 IC3.58
D33
  Top 0.254: IC3.57 76.29,41.6 96.43,21.46 96.43,13.79 97.52,12.7 CARRIERA.6
D34
  Top 0.254: IC3.56 75.82,41.1 95.9,21.02 95.9,12.42 98.16,10.16 CARRIERA.7
D35
  Top 0.203: 68.86,40.64 IC3.55
  Top 0.254: CARRIERA.8 98.03,7.62 95.25,10.4 95.25,20.67 75.28,40.64 68.86,40.64
D36
  Top 0.254: IC3.54 74.98,40.1 85.17,29.92 85.17,9.11 83.68,7.62 CARRIERA1.8
D37
  Top 0.254: IC3.53 74.57,39.6 84.75,29.43 84.75,11.36 83.55,10.16 CARRIERA1.7
D38
  Top 0.203: 82.51,17.73 82.46,17.78
  Top 0.254: IC3.50 74.86,36.6 83.37,28.09 83.37,18.59 82.51,17.73 | 82.46,17.78 CARRIERA1.4
D39
  Top 0.254: IC3.70 75.46,48.1 79.55,44.02 SV4.2
D40
  Top 0.254: CARRIERA1.6 82.79,12.7 84.28,14.19 84.28,29.08 74.26,39.1 IC3.52
D41
  Top 0.254: IC3.51 73.9,38.6 83.82,28.68 83.82,16.4 82.67,15.24 CARRIERA1.5
D42
  Top 0.203: 66.54,9.27 66.47,9.21
  Top 0.254: IC3.42 62.82,33.31 66.54,29.59 66.54,9.27 | 66.47,9.21 65.14,7.88 CARRIERA2.8
D43
  Top 0.254: IC3.41 62.32,32.92 66.03,29.21 66.03,11.43 65.01,10.42 CARRIERA2.7
D47
  Top 0.254: IC3.37 60.32,34.03 65.52,28.83 65.52,13.85 64.63,12.96 CARRIERA2.6
D48
  Top 0.254: IC3.36 59.82,33.77 65.01,28.58 65.01,16.39 64.12,15.5 CARRIERA2.5
D49
  Top 0.254: IC3.35 59.32,33.25 64.5,28.07 64.5,19.05 63.49,18.04 CARRIERA2.4
D50/MISO
  Top 0.203: ICSP.1 36.56,56.52
  Top 0.254: IC3.22 48.91,40.1 45.58,43.44 45.58,47.5 36.56,56.52
D51/MOSI
  Top 0.203: ICSP.4 39.1,63.25 37.83,61.98 37.83,56.01
  Top 0.254: IC3.21 49.27,40.6 46.09,43.78 46.09,47.75 37.83,56.01
D52/SCK
  Top 0.203: ICSP.3 39.1,55.5
  Top 0.254: IC3.20 49.44,41.1 46.6,43.95 46.6,48.01 39.1,55.5
D53/SS  (via drill 0.35)
  Top 0.254: IC3.19 50.39,41.6 v49.2,42.8
D+
  Top 0.406: Z2.2 12.14,55.32 11.88,55.32 R4.2 9.13,55.98 8.04,55.98 X2.3
D-
  Top 0.406: 12.72,50.35 R3.2 10.84,52.3 X2.2
  Top 0.508: Z1.2 12.72,50.35
DTR  (via drill 0.35, 0.41)
  Top 0.254: v22.05,53.54 IC4.13
  Top 0.305: v22.05,53.54 25.35,56.84 25.35,56.91 v25.4,56.91 26.14,57.65 C7.1
  Bottom 0.305: UBOOT.1 27.94,59.45 v25.4,56.91
GND  (via drill 0.35)
  Top 0.203: IC4.3 17.61,53.29 IC4.EXP
  Top 0.254: IC4.3 17.61,49.89
  other vias: 8.2,64.62 32.57,60.7 99.62,57.8 82.9,59.52 94.18,29.92 99.1,39.3 100.5,2.22 64.6,4.6 45.48,5.17 82.65,4.47 18.1,35.25 33.15,39.65 2.7,35.45 65.68,45.88 82.88,40.75 73.28,34.35 62.43,47.88 45.55,33 77.28,23.25 47,19.2 27.88,14.35 43.75,57.5
  pour Top: 102.1,0 102.1,67.2 0,67.2 0,0
  pour Bottom: 102.1,0 0,0 0,67.2 102.1,67.2
M8RXD
  Top 0.254: IC4.9 23.8,51.54 25.86,49.48 25.86,46.68 26.62,45.92 27.32,45.92 RN4.7
M8TXD
  Top 0.254: RN4.8 26.55,45.1 25.09,46.56 25.09,49.35 23.57,50.88 20.23,50.88 IC4.8
MISO2
  Top 0.254: IC4.17 20.11,56.49 19.76,56.84 19.76,57.86 18.87,58.75 17.73,58.75 17.09,59.38 17.09,63.32 17.6,63.83 19.12,63.83 20.27,62.69 ICSP1.1
MOSI2
  Top 0.254: IC4.16 21,55.04 21.28,55.32 21.28,56.21 20.27,57.23 20.27,58.24 ICSP1.4
N$1
  Top 1.7: U$3.P$1 12.08,6.6 12.08,10.97 9.98,13.07 J1.3
N$2
  Top 0.203: L.A 44.34,43.75 44.65,43.45 44.65,39.94 R10.1
N$3
  Top 0.254: ON.A 82.34,62.28 R11.2
N$4
  Top 1.4: U$2.P$2 26.1,22.8 23.2,19.9 23.2,14.18 26.68,10.7 D2.1
N$5
  Top 0.508: C19.2 15.91,22.12 | 11.65,22.09 IC1.2
  Top 0.61: C19.2 11.65,22.09
  Top 1.27: 17.53,22.12 19.62,20.03 C18.+ | 17.53,22.12 15.91,22.12 | U$2.P$1 20.51,25.1 17.53,22.12
N$6
  Top 0.61: C20.1 4.01,18.73 10.37,18.73 11.6,19.97 IC1.1
N$7
  Top 0.508: T2.3 8.29,38.04 R9.1 10.81,39.6 R8.2
N$8
  Top 0.508: 11.65,24.63 IC1.4
  Top 0.61: C21.2 11.65,24.63
N$9
  Top 0.508: 4.83,29.92 R7.1
  Top 0.61: 4.83,29.92 C22.1
N$10
  Top 0.813: IC1.5 7.67,25.67 R5.1 10.25,26.74 R6.2
N$11  (via drill 0.35)
  Top 0.254: IC3.49 66.37,36.56 66.37,35.57 67.04,34.9 v68.85,34.9
N$12
  Top 0.508: C22.2
  Top 0.61: C22.2 C23.2 2.5,24.45 3.54,23.41 IC1.6
N$13
  Top 0.508: C20.2 2.28,21.79 | 0.84,23.24 0.86,23.24 | 0.86,31.65 2.6,33.4 | 6.68,32.99 7.09,33.4 D8.1 7.12,33.89 13.35,40.12 21.37,40.12 22.83,38.66 22.83,34.56 L3.1
  Top 0.61: 2.28,21.79 0.84,23.24 | 0.86,23.24 0.86,31.65 | 2.6,33.4 D8.1 | IC1.8 4.75,20.87 3.82,21.79 C20.2
N$14  (via drill 0.35)
  Top 0.254: IC3.48 65.87,36.56 65.87,35.42 67.41,33.88 v70.18,33.88
N$15  (via drill 0.35)
  Top 0.254: IC3.47 65.32,35.23 67.65,32.9 68.8,32.9 v68.85,32.95
N$17  (via drill 0.35)
  Top 0.254: IC3.9 50.22,46.6 v49.8,47.02
N$18  (via drill 0.35)
  Top 0.254: IC3.8 51.34,47.1 v51.07,47.38
N$22  (via drill 0.35)
  Top 0.254: IC3.14 50.7,44.1 v50.42,44.38
N$24  (via drill 0.35)
  Top 0.254: IC3.69 74.32,47.6 v74.78,47.15
N$25  (via drill 0.35)
  Top 0.254: IC3.68 72.92,47.1 v73.15,46.88
N$26  (via drill 0.35)
  Top 0.254: IC3.67 71.67,46.6 v71.98,46.3
N$27  (via drill 0.35)
  Top 0.254: IC3.66 70.47,46.1 v70.75,45.82
N$54
  Top 0.254: RN4.4 28.69,49.01 RX.A
N$55
  Top 0.254: RN4.3 29.05,46.7 30.68,48.34 30.68,50.49 TX.A
RD+
  Top 0.305: IC4.29 13.97,53.04 12.74,54.27 R4.1
RD-
  Top 0.305: R3.1 12.93,52.54 IC4.30
RESET  (via drill 0.35)
  Top 0.203: 36.17,46.35 R12.1
  Top 0.254: IC3.30 56.82,37.6 56.45,37.98 46.49,37.98 45.49,38.98 41.97,38.98 BOUTON.1 38.8,42.15 37.77,42.15 C1.1 36.17,46.35 | R12.1 37.3,47.48 37.3,51.92 v38.09,52.71 | v41.64,56.14 ICSP.5 43.3,62.87 43.3,64.9 42.66,65.54 27.94,65.54 26.15,63.74 C7.2 28.7,62.61 RESET-EN.1
  Top 0.305: RESET-EN.1 RESET-EN.2
  Bottom 0.203: v41.64,56.14 41.52,56.14
  Bottom 0.305: 41.52,56.14 v38.09,52.71
RESET2
  Top 0.305: R13.1 23.94,62.82 22.43,64.34 16.2,64.34 15.82,63.96 ICSP1.5 14.17,61.04 14.17,59.51 16.61,57.07 IC4.24
RXL
  Top 0.254: IC4.10 24.31,52.04 RX.C
SCK2
  Top 0.254: IC4.15 21.26,54.54 21.92,55.19 21.92,56.34 20.78,57.48 20.78,58.5 19.63,59.64 19.63,61.42 ICSP1.3
TXL
  Top 0.254: IC4.11 26.35,52.54 TX.C
UGND
  Top 0.305: 14.33,57.06 14.38,57.01 14.27,56.89 14.27,54 14.74,53.54 IC4.28
  Top 0.61: L1.1 11.08,58.75 C10.2 11.16,58.33 11.94,57.53 13.84,57.53 14.33,57.06
  Top 0.813: X2.4 6.58,52.02 5.16,52.02 4.52,52.65 4.52,55.7 7.82,59 8.84,59 9.35,59.51 9.35,60.32 L1.1
  Bottom 0.813: X2.4 6.6,51.72 GROUND.1
USBVCC
  Top 0.305: IC4.31 14.45,52.04 14.3,51.89
  Top 0.406: 14.3,51.89 14.3,50.11 10.78,46.6 7.99,46.6 5.48,44.09 F1.1
  Top 0.508: F1.1 5.48,39.06 T2.1 3.12,39.01 C8.1
USHIELD  (via drill 0.41)
  Top 0.813: X2.P$2 3.88,48.21 5.16,48.21 5.79,48.84 9.78,48.84 Z1.1 | Z2.1 10.48,56.45 10.12,56.45 9.73,56.84 v9.73,57.86 | L1.2 5,60.4 X2.P$1
  Bottom 0.813: v9.73,57.86 5.57,57.86 X2.P$1
  Bottom 1.27: X2.P$2 3.88,48.21 1.98,50.11 1.98,56.46 3.88,58.37 X2.P$1
V+  (via drill 0.35)
  Top 0.508: R9.2 9.85,42.72 v10.5,43.38
  Top 1.5: D2.2 16.55,13.37 JP5.1
  Top 1.7: CARRIERB3.8 35.03,8 36.95,9.93 C29.+ | 47.46,1.3 30.23,1.3 21.39,10.14 D2.2 19.78,3.49 U$3.P$2 | 47.46,1.3 66.14,1.3 | 66.14,1.3 83.57,1.3 86.98,4.71 CARRIERB.8 90.91,7.62 93.11,9.83 C27.+ | 66.14,1.3 68.57,3.73 CARRIERB1.8 72.49,7.62 74.62,9.75 C26.+ | 47.46,1.3 49.64,3.48 CARRIERB2.8 53.82,8 C24.+
  Bottom 1.5: v10.5,43.38 13.7,40.18 13.7,15.12 15.43,13.39 JP5.1 19.33,13.37 24.7,8 CARRIERB3.8
VUCAP
  Top 0.305: IC4.27 15.2,54.04 15.19,54.05 15.19,57.35 13.92,58.62 13.24,58.62 C10.1
XT1
  Top 0.203: Q1.2 16.27,45.22 16.27,42.22
  Top 0.254: R2.1 16.27,42.22 C16.1 | IC4.1 16.61,47.89 15.85,47.12 15.85,45.7 Q1.2
XT2
  Top 0.254: R2.2 C17.1 20.85,43.95 20.85,45.61 Q1.1 20.83,45.67 17.11,49.39 IC4.2
XTAL1
  Top 0.254: IC3.34 58.82,34.63 Q2.2 C14.2 R1.1
XTAL2
  Top 0.203: 51.39,28.94 C15.2 | IC3.33 58.32,35.1
  Top 0.254: 51.39,28.94 Q2.1 53.51,34.4 57.62,34.4 58.32,35.1 | R1.2 C15.2
XVCC
  Top 0.61: F1.2 1.6,42.46 1.6,49.73 1.98,50.11 6.67,50.11 X2.1

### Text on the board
tNames: 5V MOSI GND | RESET SCK MISO | GND | GND | RX3 | TX3 | 5V | SCL | SDA | 5V | TX2 | MISO SCK RESET | A6 A7 A8 A9 A10 A11 A12 A13 A14 A15 | GND MOSI 5V | RX2 | D23 | D20 | D25 | D24 | D27 | D26 | D29 | D28 | D39 | D23 | GND | V+ GND 4B+ 4B- 4A- 4A+ +5V GND | V+ GND 3B+ 3B- 3A- 3A+ +5V GND | V+ GND 1B+ 1B- 1A- 1A+ +5V GND | A5 A4 A3 A2 A1 D2 D5 D4 | 42 43 47 48 49 3 9 6 | V+ GND 2B+ 2B- 2A- 2A+ +5V GND | 36 37 40 41 38 19 8 7 | 35 34 39 32 31 18 12 11
bNames: A+ A- B- B+ | A+ A- B- B+ | A+ A- B- B+ | A+ A- B- B+
ReferenceLC: L | TX | RX | PC1 | PC2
